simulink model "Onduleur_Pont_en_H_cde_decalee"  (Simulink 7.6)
settings: Solver=ode15s  StartTime=0.0  StopTime=2*T  RelTol=1e-3
InitFcn:
  | clear all, close all
  | clc
  | 
  | R1=1e3
  | R2=R1;
  | 
  | t1=1/9/60;
  | t2=4*t1;
  | t3=5*t1;
  | t4=8*t1;
  | t5=9*t1;
  | eps=1/90/60/1000;
  | T=9*t1;
  | 
  | R=100e3;
  | C=5/(5*pi);%2500e-3/(5*pi);%1e-3/(5*pi)
StopFcn:
  | load cde_decalee.mat
  | plot(x(1,:),x(2,:),x(1,:),x(3,:))
  | xlabel('temps')
  | title('Sinus approchée et sortie de l''onduleur')
  | grid
  | 
  | delete *.mat
libraries: powerlib x8, simulink x4

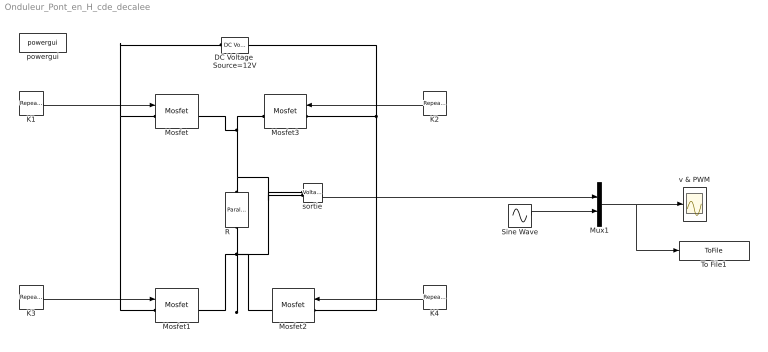
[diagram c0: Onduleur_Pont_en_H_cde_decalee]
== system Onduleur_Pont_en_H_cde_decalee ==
  DC Voltage  Source=12V : powerlib/Electrical Sources/DC Voltage Source  DialogController=POWERSYS.PowerSysDialog  SystemSampleTime=-1  Amplitude=12  Measurements=None
  K1 : simulink/Sources/Repeating Sequence  SystemSampleTime=-1  rep_seq_t=[0 t1 t1+eps t2 t2+eps t3 t3+eps t4 t4+eps t5]  rep_seq_y=[1 1 0 0 1 1 1 1 1 1]
  K2 : simulink/Sources/Repeating Sequence  SystemSampleTime=-1  rep_seq_t=[0 t1 t1+eps t2 t2+eps t3 t3+eps t4 t4+eps t5]  rep_seq_y=[0 0 1 1 0 0 0 0 0 0]
  K3 : simulink/Sources/Repeating Sequence  SystemSampleTime=-1  rep_seq_t=[0 t1 t1+eps t2 t2+eps t3 t3+eps t4 t4+eps t5]  rep_seq_y=[1 1 1 1 1 1 0 0 1 1]
  K4 : simulink/Sources/Repeating Sequence  SystemSampleTime=-1  rep_seq_t=[0 t1 t1+eps t2 t2+eps t3 t3+eps t4 t4+eps t5]  rep_seq_y=[0 0 0 0 0 0 1 1 0 0]
  Mosfet{,1..3} (4 alike) : powerlib/Power Electronics/Mosfet  DialogController=POWERSYS.PowerSysDialog  SystemSampleTime=-1  Ron=1e-6  Lon=0  Rd=0.001  Vfd=0  IC=0  Rs=1e8  Cs=inf  Measurements=on
  Mux1 : Mux  Inputs=2
  R : powerlib/Elements/Parallel RLC Branch  DialogController=POWERSYS.PowerSysDialog  PhysicalDomain=powersysdomain  SubClassName=unknown  LeftPortType=p1  RightPortType=p1  LConnTagsString=a  RConnTagsString=__new0  BranchType=R  Resistance=1e6  Inductance=1.0  SetiL0=off  InitialCurrent=0  Capacitance=25e-06  Setx0=off  InitialVoltage=0  Measurements=Branch voltage and current
  Sine Wave : Sin  Amplitude=12  Frequency=2*pi/T  SampleTime=0
  To File1 : ToFile  Filename=cde_decalee  MatrixName=x
  powergui : powerlib/powergui  SystemSampleTime=-1  SimulationMode=Continuous  SampleTime=0  frequency=60  SPID=off  DisableSnubberDevices=off  DisableRonSwitches=off  DisableVfSwitches=off  SwTol=0  Interpol=off  frequencyindice=0  echomessages=off  HookPort=off  DisplayEquations=off  FunctionMessages=off  EnableUseOfTLC=off  x0status=blocks  RestoreLinks=warning  ResistiveCurrentMeasurement=off  Frange=[0:2:500]  Ylog=off  Xlog=on  ShowGrid=off  save=off  variable=ZData  ZoomFFT=on  StartTime=0.0  cycles=1  DisplayStyle=1  fundamental=60  FreqAxis=off  MaxFrequency=1000  frequencyindicesteady=1  RmsSteady=1  display=off  Ts=0  methode=off
  sortie : powerlib/Measurements/Voltage Measurement  DialogController=POWERSYS.PowerSysDialog  SystemSampleTime=-1  PhasorSimulation=off  OutputType=Complex  PSBequivalent=0
  v & PWM : Scope
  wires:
  K1/1 -> Mosfet/1
  K2/1 -> Mosfet3/1
  K3/1 -> Mosfet1/1
  K4/1 -> Mosfet2/1
  Mux1/1 -> v & PWM/1, To File1/1
  sortie/1 -> Mux1/1
  Sine Wave/1 -> Mux1/2
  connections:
  Mosfet2/RConn1 -- Mosfet1/RConn1 -- R/RConn1 -- sortie/LConn2
  R/LConn1 -- Mosfet/RConn1 -- Mosfet3/RConn1 -- sortie/LConn1
  Mosfet1/LConn1 -- DC Voltage  Source=12V/LConn1 -- Mosfet/LConn1
  Mosfet2/LConn1 -- Mosfet3/LConn1 -- DC Voltage  Source=12V/RConn1
